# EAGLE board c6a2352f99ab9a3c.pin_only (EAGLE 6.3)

Size 26 x 40 mm. Coordinates in mm from the lower left corner, seen from the top.
Outline: 0,3 arc90 3,0 23,0 arc90 26,3 26,37 arc90 23,40 3,40 arc90 0,37 0,3
Copper layers (1*16): Top 0.035mm / dielectric 1.5mm / Bottom 0.035mm
Design rules "adafruit": minimum track width 8mil, minimum drill 15.5mil, track to track 8mil, track to pad 8mil, pad to pad 8mil, via to via 8mil, smd to smd 8mil, copper to edge 10mil, drill to drill 8mil, minimum pad ring 10mil, minimum via ring 8mil, stop-mask expansion 4mil, vias tented up to drill 20mil, thermal gap 10mil

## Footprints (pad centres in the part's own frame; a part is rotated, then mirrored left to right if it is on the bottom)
_0402 = smd 0.6 x 0.6: 1 -0.508,0; 2 0.508,0
_0805MP = smd 1.2 x 1.3: 1 -1.016,0; 2 1.016,0
FIDUCIAL_1MM = smd 1 x 1: 1 0,0
1X03_ROUND = drill 1 pad 1.676 square: 1 -2.54,0 | drill 1 pad 1.676: 2 0,0; 3 2.54,0
1X09_ROUND_70 = drill 1 pad 1.778 octagon: 1 -10.16,0 | drill 1 pad 1.778: 2 -7.62,0; 3 -5.08,0; 4 -2.54,0; 5 0,0; 6 2.54,0; 7 5.08,0; 8 7.62,0; 9 10.16,0
CHIPLED_0805_NOOUTLINE = smd 1.2 x 1.2: A 0,-1.05; C 0,1.05
0805-NO = smd 1.3 x 1.5: 1 -0.95,0; 2 0.95,0
SOLDERJUMPER_CLOSEDWIRE = smd 1.168 x 1.6: 1 -0.762,0; 2 0.762,0 | smd 0.635 x 0.203: WIRE 0,0
TESTPOINT_PAD_1MM = smd 1 x 1: P$1 0,0
CC3000MOD = smd 1.2 x 0.7: 1 -5.85,5.4; 2 -5.85,4.2; 3 -5.85,3; 4 -5.85,1.8; 5 -5.85,0.6; 6 -5.85,-0.6; 7 -5.85,-1.8; 8 -5.85,-3; 9 -5.85,-4.2; 10 -5.85,-5.4; 19 5.85,-5.4; 20 5.85,-4.2; 21 5.85,-3; 22 5.85,-1.8; 23 5.85,-0.6; 24 5.85,0.6; 25 5.85,1.8; 26 5.85,3; 27 5.85,4.2; 28 5.85,5.4 | smd 0.7 x 1.2: 11 -4.2,-7.25; 12 -3,-7.25; 13 -1.8,-7.25; 14 -0.6,-7.25; 15 0.6,-7.25; 16 1.8,-7.25; 17 3,-7.25; 18 4.2,-7.25; 29 4.2,7.25; 30 3,7.25; 31 1.8,7.25; 32 0.6,7.25; 33 -0.6,7.25; 34 -1.8,7.25; 35 -3,7.25; 36 -4.2,7.25 | smd 2.4 x 1.9: 37 -2.15,2.65; 38 -2.15,0; 39 -2.15,-2.65; 40 2.15,2.65; 41 2.15,0; 42 2.15,-2.65 | smd 1.2 x 1.2: 43 -5.85,7.25; 44 -5.85,-7.25; 45 5.85,-7.25; 46 5.85,7.25
SOT223-R = smd 1.3 x 1.3: 1 -2.3,-3.05; 2 0,-3.05; 3 2.3,-3.05 | smd 3.6 x 1.3: 4 0,3.05
SOIC16 = smd 0.6 x 2.2: 1 -4.445,-2.6; 2 -3.175,-2.6; 3 -1.905,-2.6; 4 -0.635,-2.6; 5 0.635,-2.6; 6 1.905,-2.6; 7 3.175,-2.6; 8 4.445,-2.6; 9 4.445,2.6; 10 3.175,2.6; 11 1.905,2.6; 12 0.635,2.6; 13 -0.635,2.6; 14 -1.905,2.6; 15 -3.175,2.6; 16 -4.445,2.6
MOUNTINGHOLE_2.5_PLATED = drill 2.5 pad 3.2: P$1 0,0
U.FL = smd 2.2 x 0.85: P$1 0,1.375; P$2 0,-1.375 | smd 1.05 x 1: P$3 1.525,0; P$4 -1.525,0
ANT_2500AT44M0400 = smd 1 x 1.5: FEED 4,0; NC -4,0

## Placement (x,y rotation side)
C1  2.2pF  [_0402]  13.65,36 0 top
C2  10pF  [_0402]  10,32.5 270 top
C3  DNC_10pF  [_0402]  9.5,32 180 top
C4  1µF  [_0805MP]  22,21.5 90 top
C5  1µF  [_0805MP]  22,16.6 90 top
C6  10µF  [_0805MP]  11.5,5.4 90 top
C7  10µF  [_0805MP]  2.5,4.7 180 top
C8  10µF  [_0805MP]  2.5,11.3 180 top
FB1  [_0805MP]  11.5,10.2 90 top
FID1  FIDUCIAL""  [FIDUCIAL_1MM]  19.05,31.75 0 top
FID2  FIDUCIAL""  [FIDUCIAL_1MM]  1.52,7.62 0 top
FID3  FIDUCIAL""  [FIDUCIAL_1MM]  1.52,31.75 0 top
JP1  [1X03_ROUND]  2.29,20.45 270 top
JP3  [1X09_ROUND_70]  13,2 180 top
L1  DNP  [_0402]  15.39,35.5 90 top
L2  2.2nH  [_0402]  11.9,35.5 90 top
LED1  green  [CHIPLED_0805_NOOUTLINE]  2.54,13.72 90 top
R1  470  [0805-NO]  2.54,15.62 180 top
R2  10K  [_0805MP]  24.5,6.8 90 top
R3  10K  [_0805MP]  23,13.9 0 top
SJ1  TESTMODE  [SOLDERJUMPER_CLOSEDWIRE]  9,20.5 90 bottom
TP1  SCL  [TESTPOINT_PAD_1MM]  16.5,24 0 bottom
TP2  SDA  [TESTPOINT_PAD_1MM]  16.5,21.5 0 bottom
U1  CC3000MOD  [CC3000MOD]  13,21 0 top
U2  [SOT223-R]  6.5,8 90 top
U3  74HC4050D  [SOIC16]  18.03,7.62 0 top
U$8  [ADAFRUIT_5MM]  21.07,29.18 0 top
U$24  MOUNTINGHOLE2.5  [MOUNTINGHOLE_2.5_PLATED]  2.5,26.5 0 top
U$34  MOUNTINGHOLE2.5  [MOUNTINGHOLE_2.5_PLATED]  23.5,26.5 0 top
U$35  U.FL  [U.FL]  5,36 270 top
U$36  [ADAFRUIT_TEXT_20MM]  24.13,27.18 0 bottom
X1  2500AT44M0400E  [ANT_2500AT44M0400]  20.69,36 180 top

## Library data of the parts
C1-C8 FB1 L1 L2 LED1 R1-R3 SJ1 TP1 TP2 U1-U3 U$8 U$35 U$36 X1 = microbuilder
FID1 FID2 U$24 U$34 = microbuilder; BOM: EXCLUDE
FID3 = microbuilder; BOM: EXCLUDE; COMPANY: ADAFRUIT INDUSTRIES; DRAWN: KTOWN; REV: C
JP1 JP3 = microbuilder; COMPANY: ADAFRUIT INDUSTRIES; DRAWN: KTOWN; REV: C

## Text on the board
tPlace: Adafruit CC3000 WiFi | GND | TXD | Debug | RXD | GND | VIN | MISO | CS | IRQ | 3V3 | CLK | MOSI | VBEN
bPlace: Test | Adafruit CC3000 WiFi / 802.11b/g / SPI Interface | Vin: 3-5VDC / Logic: 3-5VDC

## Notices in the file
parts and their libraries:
microbuilder: This work is placed in the public domain, and may be freely used for commercial and non-commercial work with the following conditions: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
